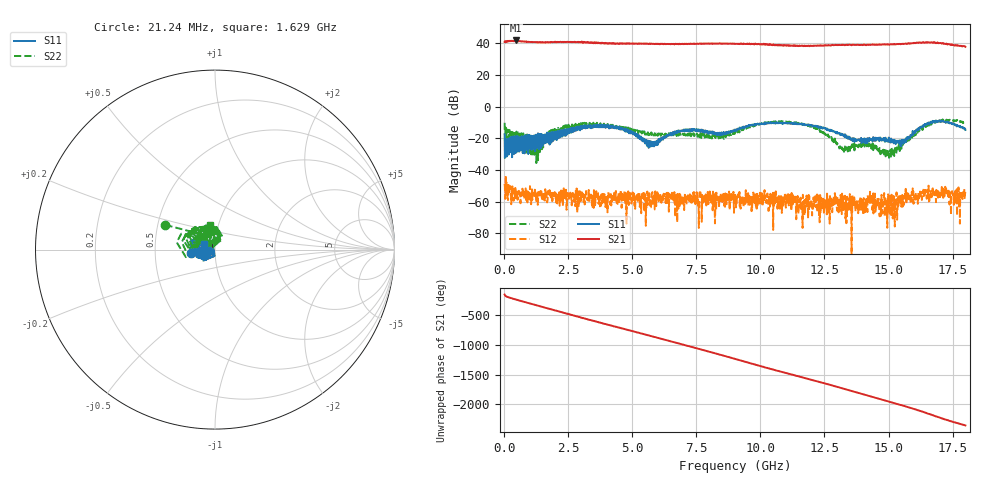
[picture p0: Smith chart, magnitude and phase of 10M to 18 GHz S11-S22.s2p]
!Agilent Technologies,E8361C,US49010292,A.09.42.06
!Agilent E8361C: A.09.42.06
!Date: Wednesday, May 21, 2025 00:38:07
!Correction: S11(Full 2 Port(1,2))
!S21(Full 2 Port(1,2))
!S12(Full 2 Port(1,2))
!S22(Full 2 Port(1,2))
!S2P File: Measurements: S11, S21, S12, S22:
# Hz S  dB  R 50
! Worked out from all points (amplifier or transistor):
!   1600 points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, 21.24 MHz to 18 GHz, reference 50 ohm
!   highest |S21| = 41.8 dB at 448.5 MHz (marker M1)
!   |S21| within 3 dB of that: start of sweep to 10.54 GHz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
!   unconditionally stable (mu >= 1): start of sweep to end of sweep
!   at 3.012 GHz: K = 3.76, MAG = 41.3 dB, |S12| = -59.2 dB
!   at 9.016 GHz: K = 3.77, MAG = 40.0 dB, |S12| = -57.6 dB
!   at 18 GHz: K = 2.64, MAG = 38.5 dB, |S12| = -53.3 dB
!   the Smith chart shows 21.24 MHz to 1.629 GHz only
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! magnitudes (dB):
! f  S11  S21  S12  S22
! 21.24 MHz  -17.4  40.9  -48.8  -10.2
! 448.5 MHz  -29.4  41.8  -53.7  -23.8
! 1.247 GHz  -17.7  40.7  -54.2  -25.0
! 2.113 GHz  -18.4  40.8  -58.9  -13.4
! 3.023 GHz  -13.0  41.0  -57.3  -11.4
! 4.418 GHz  -12.8  39.8  -60.0  -13.4
! 5.643 GHz  -26.0  39.6  -58.7  -18.0
! 6.014 GHz  -21.5  39.6  -56.6  -17.1
! 7.071 GHz  -14.4  39.6  -54.8  -17.9
! 9.016 GHz  -15.4  39.8  -57.6  -16.0
! 10.51 GHz  -10.3  39.4  -52.9  -9.4
! 12.01 GHz  -12.1  38.6  -61.0  -12.7
! 13.2 GHz  -17.7  39.2  -59.8  -26.5
! 14.12 GHz  -21.8  38.9  -59.0  -23.6
! 14.31 GHz  -21.0  39.1  -57.4  -24.5
! 14.73 GHz  -21.5  39.3  -55.7  -29.1
! 15.01 GHz  -19.5  39.3  -62.4  -29.3
! 15.2 GHz  -23.2  39.5  -56.4  -27.7
! 15.56 GHz  -23.4  39.8  -56.5  -24.2
! 16.77 GHz  -9.0  40.9  -55.8  -9.7
! 17.76 GHz  -12.4  38.4  -55.8  -9.3
! 18 GHz  -14.7  37.8  -53.3  -10.0
